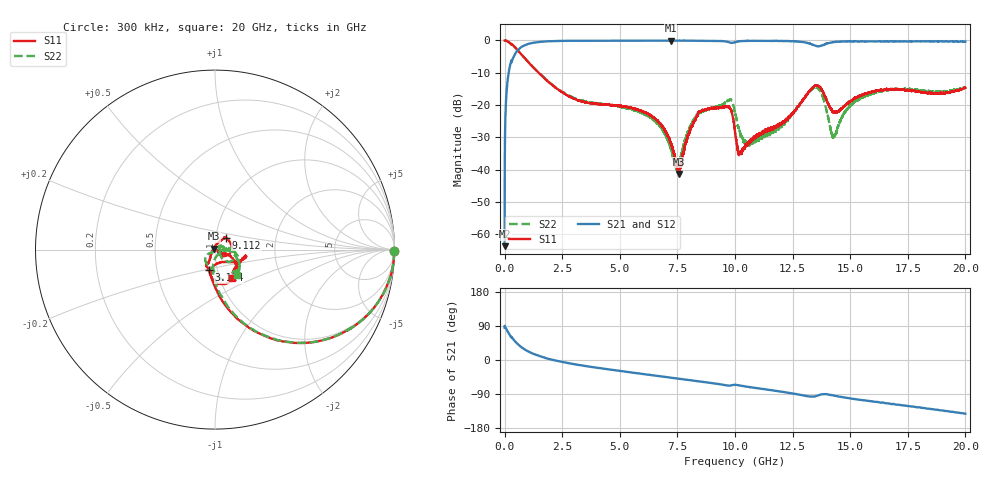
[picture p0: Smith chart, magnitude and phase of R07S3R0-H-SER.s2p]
!{R07S3R0}
!Johanson Technology Inc.
!www.johansontechnology.com
!Test Board Conditions:
!Substrate Type  RO4350B
!Substrate Thickness  10 mil
!Substrate Dk  3.66
!TL Type: GCPW
!TL Trace Width  21 mil
!TL Gap  20 mil
!Electrode orientation  Horizontal
!DUT TOPOLOGY	SERIES
!Mounting Pad LxW  16x21 mil
! Created Sat Feb  6 11:30:05 2021
# hz S ma R 50
! 2 Port Network Data from SP1.SP block
! freq  magS11  angS11  magS21  angS21  magS12  angS12  magS22  angS22
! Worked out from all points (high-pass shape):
!   20001 points, 300 kHz to 20 GHz, reference 50 ohm
!   highest |S21| = -0.03 dB at 7.201 GHz (marker M1); lowest = -63.7 dB at 300 kHz (marker M2)
!   |S21| within 3 dB of the highest: 569.2 MHz to end of sweep
!   lowest |S11| = -41.4 dB at 7.564 GHz (marker M3), VSWR 1.02, Z = 49.3 + j0.494 ohm
!   |S11| at or under -10 dB: 1.475 GHz to end of sweep
!   |S22| runs from -40.3 to 0.0 dB; largest |S21 - S12| = 0.012
!   S11 on the Smith chart (normalised r, x): 300 kHz: open; 3.124 GHz: 0.91, -0.21; 9.112 GHz: 1.12, +0.15; 20 GHz: 1.14, -0.38
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300000  0.998 -0.4  0.0006501 84.9  0.0006623 92.1  1 -0.5
1.263e8  0.9711 -14.2  0.234 76.1  0.2339 76.1  0.971 -14.2
4.293e8  0.7975 -38.7  0.5964 50.9  0.5953 51.0  0.7984 -38.6
1.2883e9  0.3682 -74.9  0.9259 15.4  0.9262 15.3  0.3716 -73.8
3.1243e9  0.1203 -106.5  0.9893 -12.1  0.9888 -12.1  0.1237 -94.9
3.3343e9  0.1142 -109.3  0.9898 -14.2  0.9891 -14.2  0.1177 -95.8
6.6673e9  0.05596 -119.4  0.9948 -42.2  0.995 -42.3  0.05055 -145.7
7.2013e9  0.02633 -134.9  0.9965 -46.6  0.9947 -46.5  0.02246 -137.1
7.5643e9  0.008546 144.1  0.9946 -49.5  0.9931 -49.5  0.01211 -43.5
8.3853e9  0.06898 54.1  0.9899 -56.0  0.9901 -56.0  0.07375 6.2
9.1123e9  0.09043 47.6  0.9849 -62.0  0.9854 -62.0  0.09014 0.7
9.7603e9  0.09128 0.2  0.9354 -67.6  0.935 -67.7  0.1194 -18.0
1.00003e10  0.03882 -46.9  0.9413 -65.4  0.9403 -65.6  0.07567 -50.5
1.02103e10  0.01777 -15.9  0.9734 -67.2  0.9726 -67.3  0.0381 -38.9
1.07003e10  0.02785 -16.6  0.9865 -72.1  0.9852 -72.1  0.02671 15.5
1.20823e10  0.05489 -25.3  0.9806 -84.2  0.9807 -84.3  0.0507 14.9
1.33343e10  0.1814 -50.9  0.8698 -96.6  0.8701 -96.6  0.1755 -39.9
1.37303e10  0.1801 -89.5  0.8282 -91.0  0.8252 -91.0  0.1564 -82.0
1.42913e10  0.0776 -79.6  0.9437 -93.9  0.9448 -93.9  0.03246 -43.8
1.52073e10  0.1296 -32.8  0.9736 -103.0  0.9702 -102.9  0.1159 -9.0
1.66673e10  0.1708 -13.4  0.9587 -114.6  0.9641 -114.9  0.1722 -41.6
2e10  0.1842 -60.0  0.9621 -141.7  0.9569 -141.6  0.1877 -48.4
